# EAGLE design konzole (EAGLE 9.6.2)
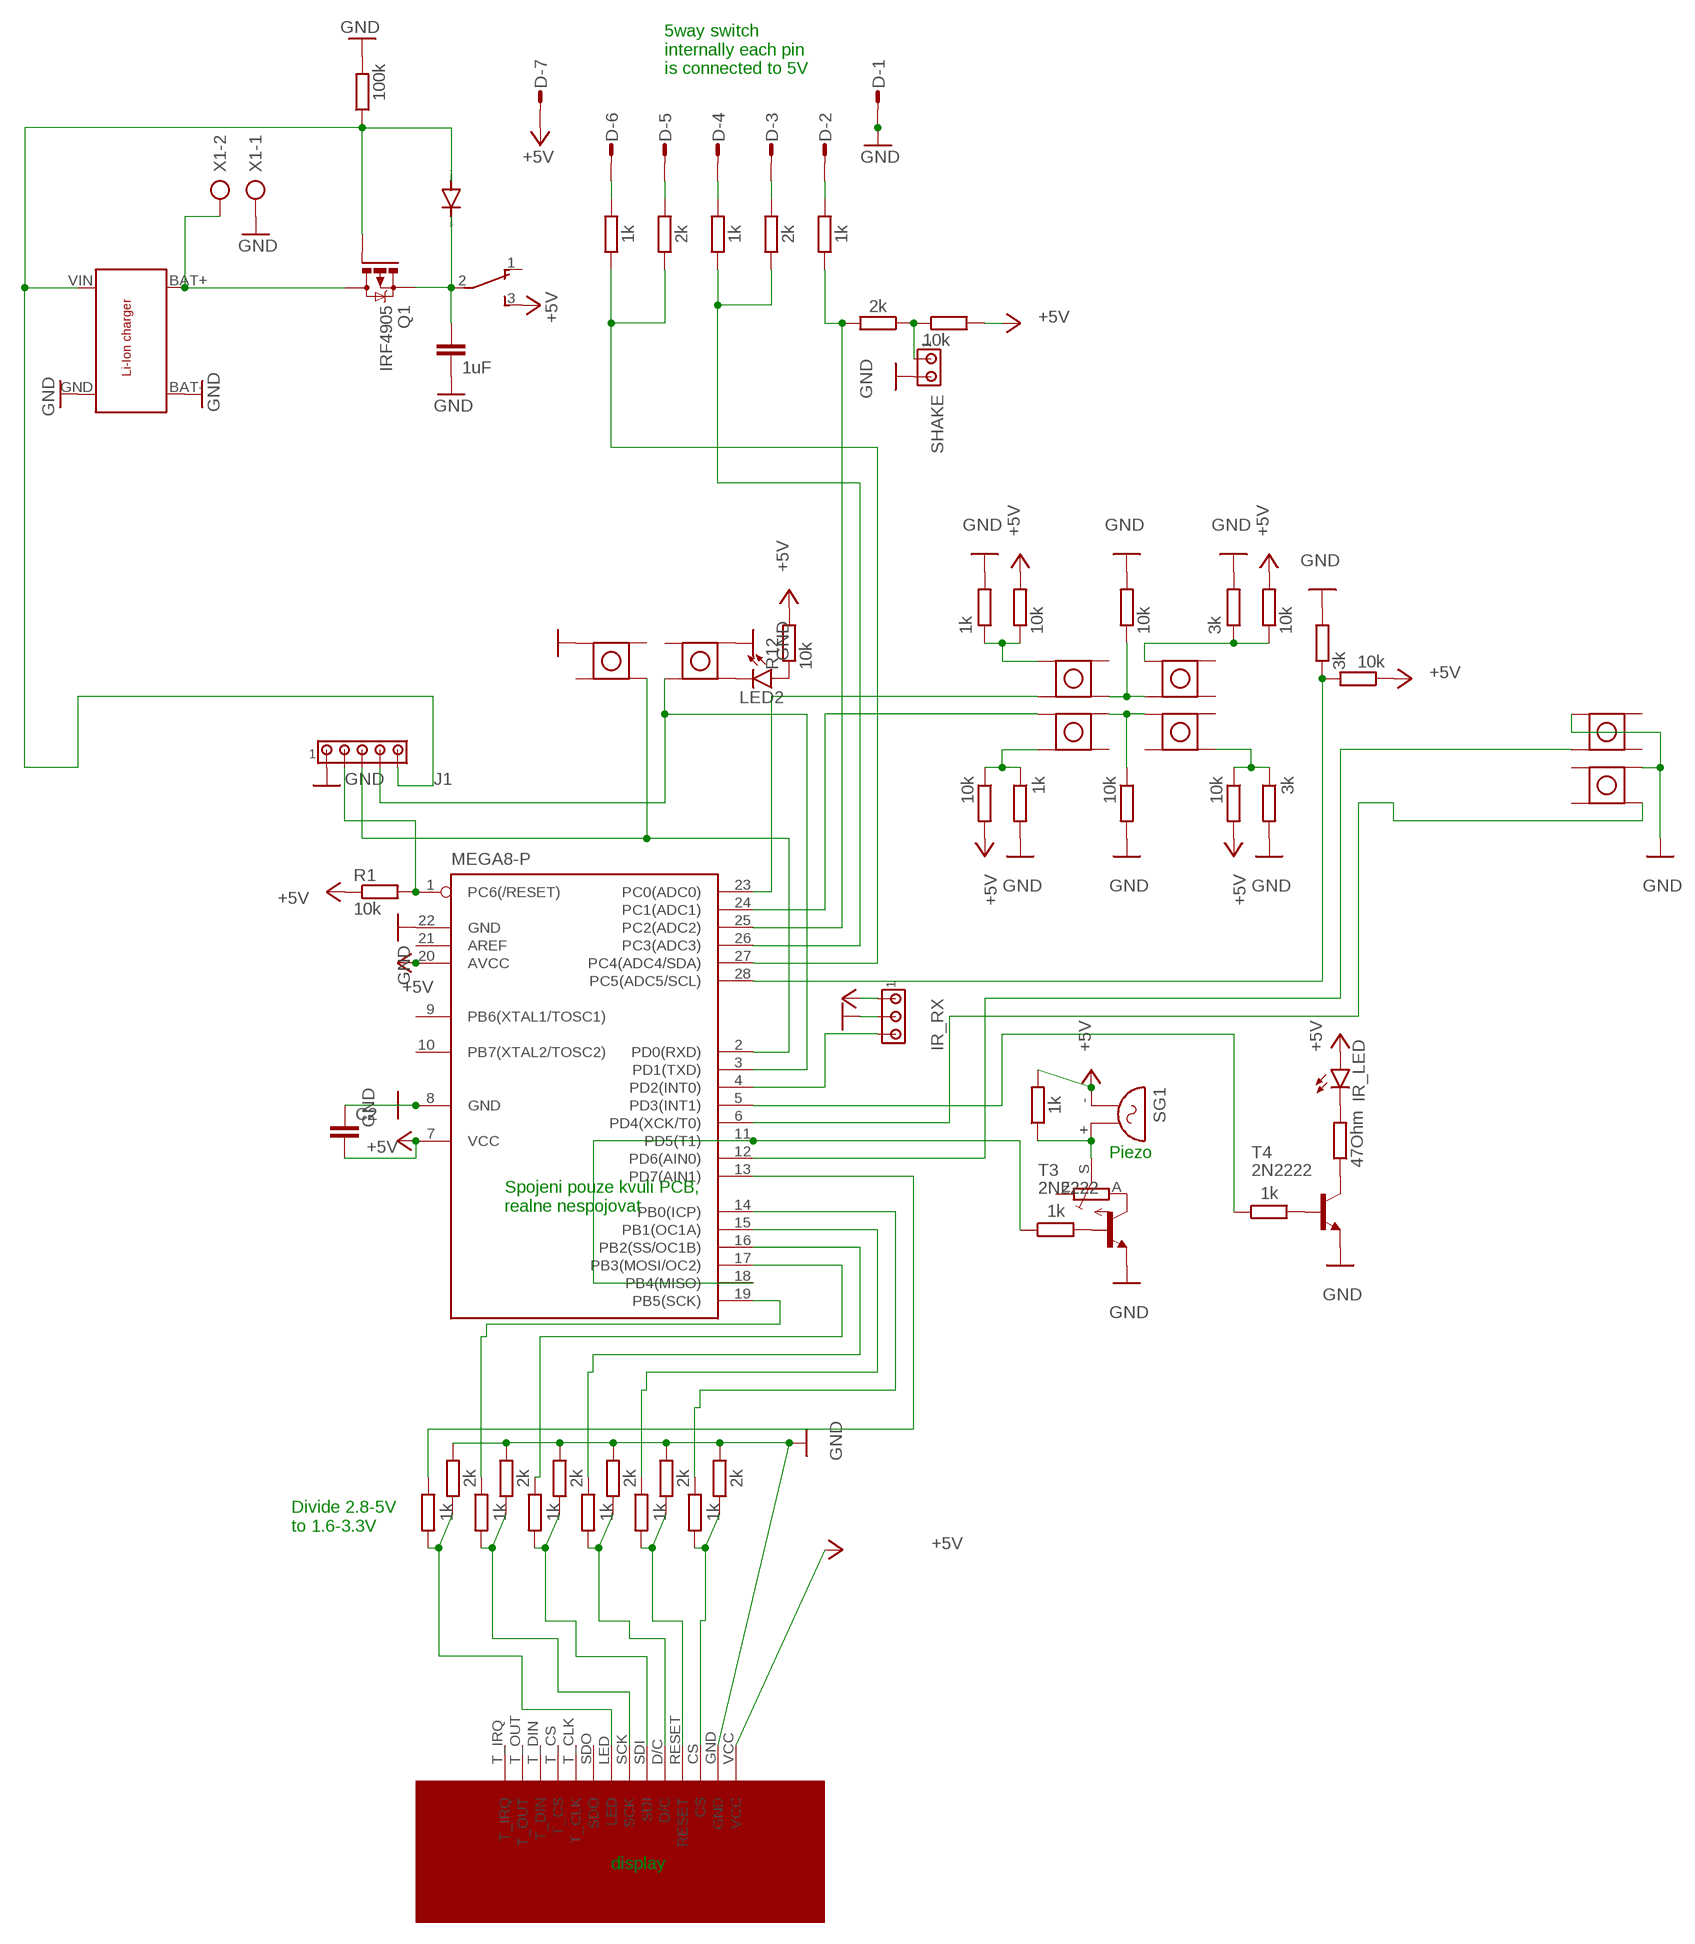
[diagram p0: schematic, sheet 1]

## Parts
C1  1uF  C-EU050-025X075  [C050-025X075]
C2  C5/2.5  [C5B2.5]
D  L07P  [L07P]
D1  1N4004  [DO41-10]
IC1  MEGA8-P  [DIL28-3]
IR_LED  LED5MM  [LED5MM]
IR_RX  MTA03-100  [10X03MTA]
J1  MTA05-100  [10X05MTA]
LED2  LED3MM  [LED3MM]
Q1  IRF4905  [TO220BH]
R1  10k  R-EU_0207/10  [0207/10]
R2  1k  R-EU_0207/10  [0207/10]
R3  2k  R-EU_0207/10  [0207/10]
R4  1k  R-EU_0207/10  [0207/10]
R5  2k  R-EU_0207/10  [0207/10]
R6  1k  R-EU_0207/10  [0207/10]
R7  2k  R-EU_0207/10  [0207/10]
R8  1k  R-EU_0207/10  [0207/10]
R9  2k  R-EU_0207/10  [0207/10]
R10  1k  R-EU_0207/10  [0207/10]
R11  2k  R-EU_0207/10  [0207/10]
R12  10k  R-EU_0207/10  [0207/10]
R13  3k  R-EU_0207/10  [0207/10]
R14  10k  R-EU_0207/10  [0207/10]
R15  1k  R-EU_0207/10  [0207/10]
R16  10k  R-EU_0207/10  [0207/10]
R17  3k  R-EU_0207/10  [0207/10]
R18  10k  R-EU_0207/10  [0207/10]
R19  1k  R-EU_0207/10  [0207/10]
R20  10k  R-EU_0207/10  [0207/10]
R21  3k  R-EU_0207/10  [0207/10]
R22  10k  R-EU_0207/10  [0207/10]
R23  10k  R-EU_0207/10  [0207/10]
R24  1k  R-EU_0207/10  [0207/10]
R25  2k  R-EU_0207/10  [0207/10]
R26  1k  R-EU_0207/10  [0207/10]
R27  1k  R-EU_0207/10  [0207/10]
R28  TRIM_EU-CIP20C-6MM  [CIP20C-6MM]
R29  10k  R-EU_0207/10  [0207/10]
R33  1k  R-EU_0207/10  [0207/10]
R34  47Ohm  R-EU_0207/10  [0207/10]
R35  1k  R-EU_0207/10  [0207/10]
R36  2k  R-EU_0207/10  [0207/10]
R38  1k  R-EU_0207/10  [0207/10]
R39  2k  R-EU_0207/10  [0207/10]
R40  1k  R-EU_0207/10  [0207/10]
R41  2k  R-EU_0207/10  [0207/10]
R42  100k  R-EU_0207/10  [0207/10]
R49  10k  R-EU_0207/10  [0207/10]
S1  TL36PO  [TL3XPO]
SG1  F/QMX  [F/QMX]
SHAKE  MTA02-100  [10X02MTA]
T3  2N2222  [TO92-EBC-OVAL]
T4  2N2222  [TO92-EBC-OVAL]
U$1  TACT  [TACT]
U$2  DISPLAY  [DISPLAY]
U$3  TACT  [TACT]
U$4  TACT  [TACT]
U$5  TACT  [TACT]
U$6  TACT  [TACT]
U$7  TACT  [TACT]
U$8  TACT  [TACT]
U$9  TACT  [TACT]
U$10  LI_ION_CHARGER  [LI_ION_CHARGER]
X1  AK500/2  [AK500/2]

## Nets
+5V: C2.2 D.7 IC1.7(VCC) IC1.20(AVCC) IR_LED.A IR_RX.1 R1.1 R12.2 R14.2 R16.2 R18.2 R20.2 R27.2 R29.1 R49.2 S1.3(S) SG1.- U$2.VCC
GND: C1.2 C2.1 D.1 IC1.8(GND) IC1.22(GND) IR_RX.2 J1.1 R3.2 R5.2 R7.2 R9.2 R11.2 R13.2 R15.2 R17.2 R19.2 R21.2 R22.2 R23.2 R25.2 R42.2 SHAKE.2 T3.E T4.E U$2.GND U$6.P$4 U$7.P$1 U$8.P$1 U$9.P$4 U$10.BAT- U$10.GND X1.1
N$1: IC1.1(PC6(/RESET)) J1.2 R1.2
N$2: R2.2 R3.1 U$2.CS
N$3: R4.2 R5.1 U$2.RESET
N$4: R6.2 R7.1 U$2.D/C
N$5: R8.2 R9.1 U$2.SDI
N$6: R10.2 R11.1 U$2.SCK
N$7: IC1.17(PB3(MOSI/OC2)) R8.1
N$8: IC1.13(PD7(AIN1)) R24.1
N$9: IC1.16(PB2(SS/OC1B)) R6.1
N$10: IC1.15(PB1(OC1A)) R4.1
N$11: R14.1 R15.1 U$1.P$1
N$12: R27.1 R28.S SG1.+
N$13: IC1.19(PB5(SCK)) R10.1
N$14: R16.1 R17.1 U$5.P$1
N$15: R18.1 R19.1 U$3.P$2
N$16: R20.1 R21.1 U$4.P$3
N$17: R33.2 T4.B
N$18: LED2.K(C) U$9.P$3
N$19: IC1.2(PD0(RXD)) J1.3 U$8.P$3
N$20: IC1.3(PD1(TXD)) J1.4 U$9.P$2
N$21: R23.1 U$3.P$4 U$4.P$1
N$22: R22.1 U$1.P$3 U$5.P$2
N$23: IC1.23(PC0(ADC0)) U$1.P$2
N$24: R24.2 R25.1 U$2.LED
N$25: IC1.24(PC1(ADC1)) U$3.P$1
N$26: R34.1 T4.C
N$27: IC1.11(PD5(T1)) IC1.18(PB4(MISO)) R26.1
N$28: R26.2 T3.B
N$29: R28.A T3.C
N$30: IC1.14(PB0(ICP)) R2.1
N$32: IC1.12(PD6(AIN0)) U$7.P$2
N$33: IC1.28(PC5(ADC5/SCL)) R13.1 R29.2
N$34: IC1.6(PD4(XCK/T0)) U$6.P$3
N$35: LED2.A R12.1
N$36: IC1.4(PD2(INT0)) IR_RX.3
N$39: IR_LED.K(C) R34.2
N$40: IC1.5(PD3(INT1)) R33.1
N$41: D.6 R38.2
N$42: D.5 R36.2
N$43: D.4 R35.2
N$44: Q1.D U$10.BAT+ X1.2
N$45: D.3 R39.2
N$46: D.2 R40.2
N$48: IC1.26(PC3(ADC3)) R35.1 R39.1
N$49: R41.1 R49.1 SHAKE.1
N$50: D1.A J1.5 Q1.G R42.1 U$10.VIN
N$51: C1.1 D1.C Q1.S S1.2(P)
N$52: IC1.25(PC2(ADC2)) R40.1 R41.2
N$54: IC1.27(PC4(ADC4/SDA)) R36.1 R38.1
Unconnected: IC1.9(PB6(XTAL1/TOSC1)) IC1.10(PB7(XTAL2/TOSC2)) IC1.21(AREF) R28.E S1.1(O) U$1.P$4 U$2.SDO U$2.T_CLK U$2.T_CS U$2.T_DIN U$2.T_IRQ U$2.T_OUT U$3.P$3 U$4.P$2 U$4.P$4 U$5.P$3 U$5.P$4 U$6.P$1 U$6.P$2 U$7.P$3 U$7.P$4 U$8.P$2 U$8.P$4 U$9.P$1

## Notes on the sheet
- 5way switch
  internally each pin
  is connected to 5V
- Piezo
- Spojeni pouze kvuli PCB, 
  realne nespojovat
- Divide 2.8-5V
  to 1.6-3.3V
- display

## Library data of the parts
C1 = rcl:C-EU: CAPACITOR, European symbol; SPICEPREFIX: C
C2 = capacitor-wima:C: CAPACITOR
D = con-amp-mt:L07P: AMP MT CONNECTOR; OC_FARNELL: unknown; OC_NEWARK: unknown
D1 = diode:1N4004: DIODE
IC1 = atmel:MEGA8-P: MICROCONTROLLER 8 Kbytes FLASH, 1 kbytes SRAM, 512 bytes EEPROM, USART, 4-channel 10 bit ADC, 2-channel 8 bit ADC Pin compatible with Atmega48, ATMega88, ATMega168 Source: avr.lbr; OC_FARNELL: unknown; OC_NEWARK: unknown
IR_LED LED2 = led:LED: LED
IR_RX = con-amp:MTA03-100: AMP connector
J1 = con-amp:MTA05-100: AMP connector
Q1 = transistor-power:IRF4905: P-Channel HEXFET® Power MOSFET RDS(on)= 0.02 Ohm, ID = -74A Source: http://www.irf.com/product-info/datasheets/data/irf4905pbf.pdf
R1-R27 R29 R33-R36 R38-R42 R49 = rcl:R-EU_: RESISTOR, European symbol; SPICEPREFIX: R
R28 = pot:TRIM_EU-: POTENTIOMETER
S1 = switch:TL36PO: TINY SWITCH ON - ON Source: http://www2.produktinfo.conrad.com/datenblaetter/700000-724999/705152-da-01-de-Subminiaturschalter_TL_36YO.pdf
SG1 = buzzer:F/QMX: BUZZER; OC_FARNELL: unknown; OC_NEWARK: unknown
SHAKE = con-amp:MTA02-100: AMP connector
T3 T4 = adafruit:2N2222: NPN TRANSISTOR Big oval pads
U$1 U$3-U$9 = PSicho:TACT
U$2 = PSicho:DISPLAY
U$10 = PSicho:LI_ION_CHARGER
X1 = con-ptr500:AK500/2: CONNECTOR; OC_FARNELL: unknown; OC_NEWARK: unknown

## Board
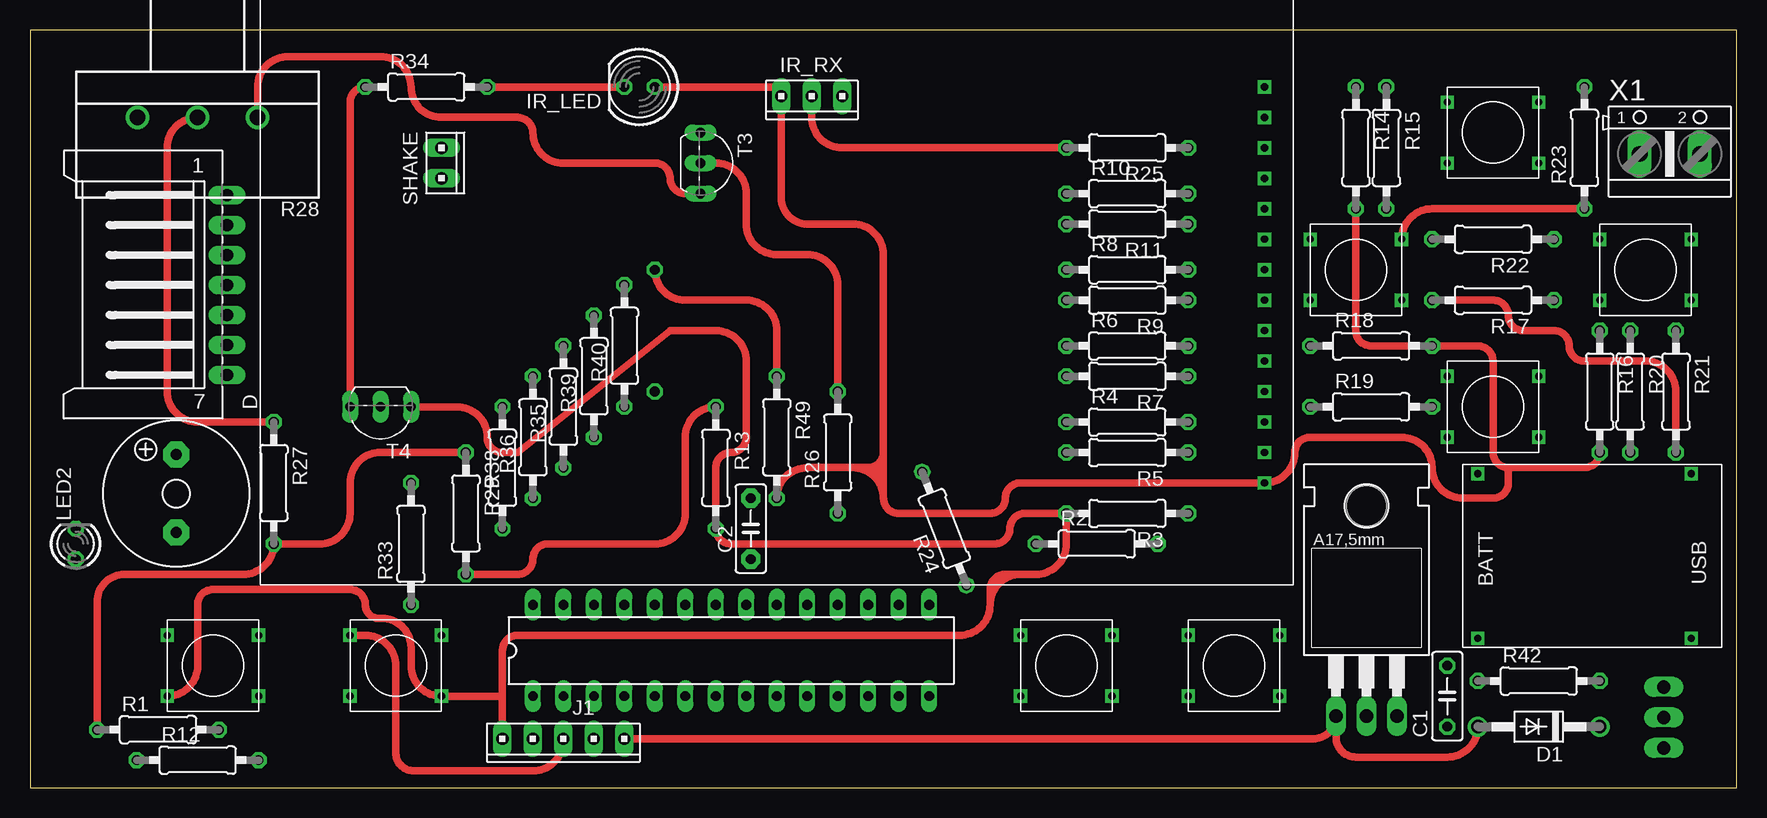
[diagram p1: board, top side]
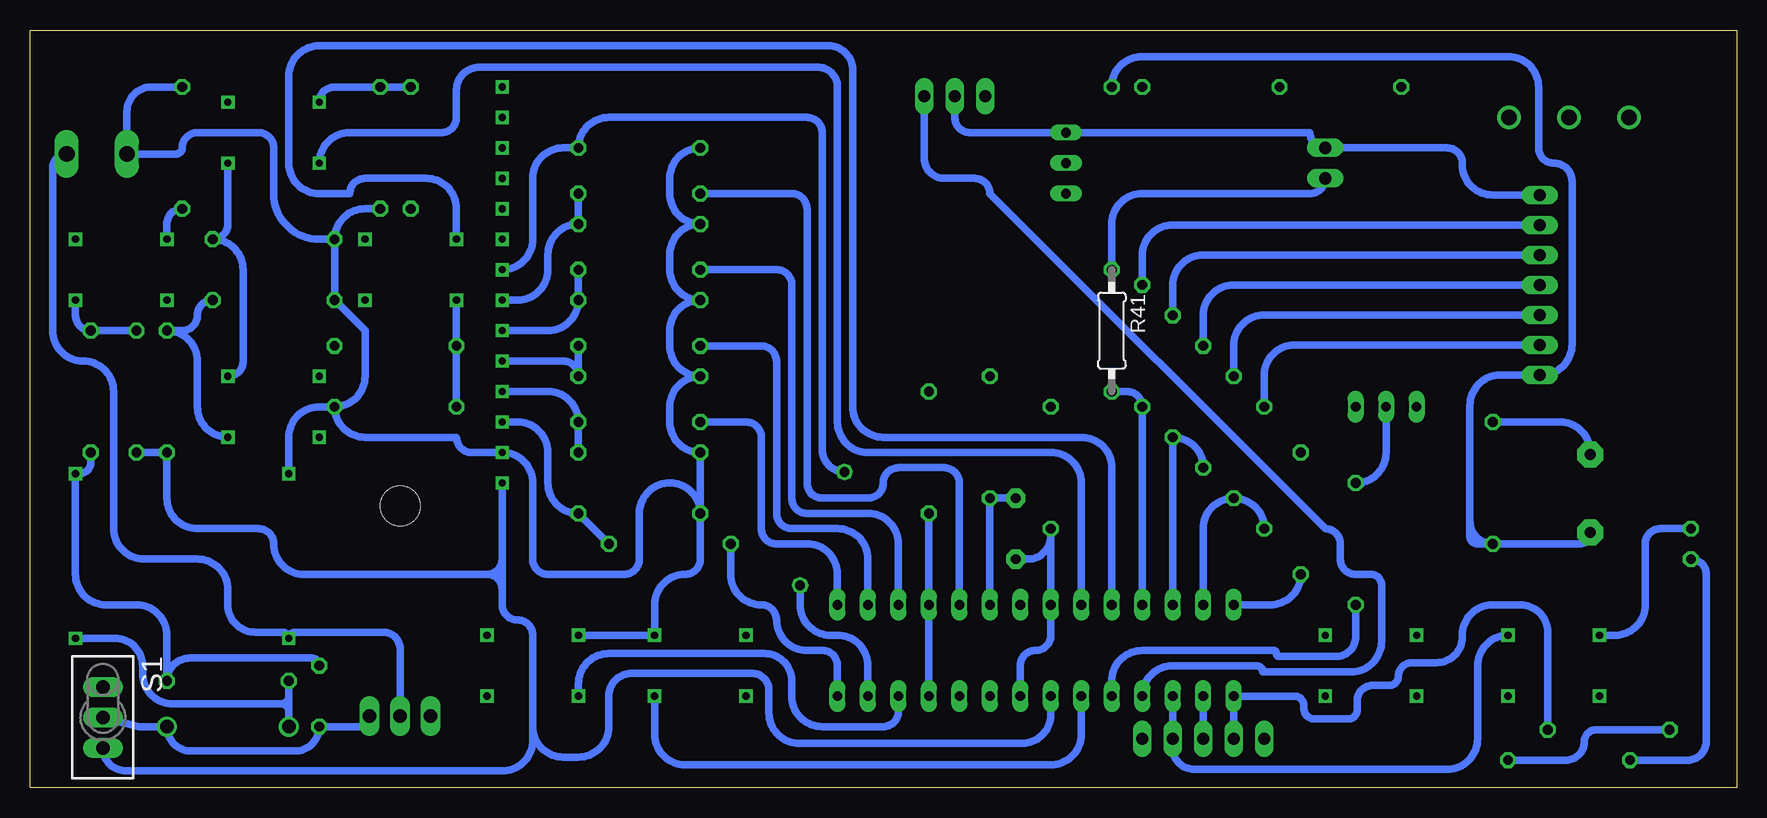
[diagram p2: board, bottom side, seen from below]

Size 142.22 x 63.17 mm. Coordinates in mm from the lower left corner, seen from the top.
Outline: 0,0 142.22,0 142.22,63.17 0,63.17 0,0
Copper layers (1*16): Top 0.035mm / dielectric 1.5mm / Bottom 0.035mm
Design rules "default *": minimum track width 24mil, minimum drill 0.6mm, track to track 24mil, track to pad 24mil, pad to pad 24mil, via to via 24mil, smd to smd 6mil, copper to edge 40mil, drill to drill 6mil, minimum pad ring 10mil, minimum via ring 8mil, stop-mask expansion 4mil, vias tented up to drill 0mil, thermal gap 10mil

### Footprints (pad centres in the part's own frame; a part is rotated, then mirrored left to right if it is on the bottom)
C050-025X075 = drill 0.813 octagon: 1 -2.54,0; 2 2.54,0
C5B2.5 = drill 0.813 pad 1.6 octagon: 1 -2.54,0; 2 2.54,0
L07P = drill 1.016 long: 1 7.5,-6.25; 2 5,-6.25; 3 2.5,-6.25; 4 0,-6.25; 5 -2.5,-6.25; 6 -5,-6.25; 7 -7.5,-6.25
DO41-10 = drill 1.118: A 5.08,0; C -5.08,0
DIL28-3 = drill 0.813 long: 1 -16.51,-3.81; 2 -13.97,-3.81; 3 -11.43,-3.81; 4 -8.89,-3.81; 5 -6.35,-3.81; 6 -3.81,-3.81; 7 -1.27,-3.81; 8 1.27,-3.81; 9 3.81,-3.81; 10 6.35,-3.81; 11 8.89,-3.81; 12 11.43,-3.81; 13 13.97,-3.81; 14 16.51,-3.81; 15 16.51,3.81; 16 13.97,3.81; 17 11.43,3.81; 18 8.89,3.81; 19 6.35,3.81; 20 3.81,3.81; 21 1.27,3.81; 22 -1.27,3.81; 23 -3.81,3.81; 24 -6.35,3.81; 25 -8.89,3.81; 26 -11.43,3.81; 27 -13.97,3.81; 28 -16.51,3.81
LED5MM = drill 0.813 octagon: A -1.27,0; K 1.27,0
10X03MTA = drill 1.016 long: 1 2.54,0; 2 0,0; 3 -2.54,0
10X05MTA = drill 1.016 long: 1 5.08,0; 2 2.54,0; 3 0,0; 4 -2.54,0; 5 -5.08,0
LED3MM = drill 0.813 octagon: A -1.27,0; K 1.27,0
TO220BH = drill 1.118 long: D 0,-6.35; G -2.54,-6.35; S 2.54,-6.35 | hole 3.302: 0,11.176
0207/10 = drill 0.813 octagon: 1 -5.08,0; 2 5.08,0
CIP20C-6MM = drill 1.3 pad 1.93: A -5,0; E 5,0; S 0,0
TL3XPO = drill 1.1 pad 1.422 long: 1 -2.54,0; 2 0,0; 3 2.54,0
F/QMX = drill 0.914 pad 2.159 octagon: + 3.251,0; - -3.251,0
10X02MTA = drill 1.016 long: 1 1.27,0; 2 -1.27,0
TO92-EBC-OVAL = drill 0.813 long: B 0,-1.27; C 2.54,-1.27; E -2.54,-1.27
TACT = drill 0.6 square: P$1 -3.81,2.54; P$2 -3.81,-2.54; P$3 3.81,-2.54; P$4 3.81,2.54
DISPLAY = drill 0.6 square: CS -40.64,11.43; D/C -40.64,6.35; GND -40.64,13.97; LED -40.64,-1.27; RESET -40.64,8.89; SCK -40.64,1.27; SDI -40.64,3.81; SDO -40.64,-3.81; T_CLK -40.64,-6.35; T_CS -40.64,-8.89; T_DIN -40.64,-11.43; T_IRQ -40.64,-16.51; T_OUT -40.64,-13.97; VCC -40.64,16.51
LI_ION_CHARGER = drill 0.6 square: BAT+ 8.89,6.858; BAT- 8.89,-6.858; GND -8.89,-6.858; VIN -8.89,6.858
AK500/2 = drill 1.321 long: 1 -2.515,0; 2 2.515,0

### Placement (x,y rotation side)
C1  118.11,7.62 90 top
C2  60.07,21.59 90 top
D  10.16,41.91 90 top
D1  125.73,5.08 180 top
IC1  58.42,11.43 0 top
IR_LED  50.8,58.42 180 top
IR_RX  65.15,57.66 180 top
J1  44.45,4.06 180 top
LED2  3.81,20.32 90 top
Q1  111.38,12.32 0 top
R1  10.67,4.83 0 top
R2  88.9,20.32 0 top
R3  91.44,22.86 180 top
R4  91.44,30.48 0 top
R5  91.44,27.94 180 top
R6  91.44,36.83 0 top
R7  91.44,34.29 180 top
R8  91.44,43.18 0 top
R9  91.44,40.64 180 top
R10  91.44,49.53 0 top
R11  91.44,46.99 180 top
R12  13.97,2.29 0 top
R13  57.15,26.67 270 top
R14  110.49,53.34 270 top
R15  113.03,53.34 270 top
R16  130.81,33.02 270 top
R17  121.92,40.64 180 top
R18  111.76,36.83 0 top
R19  111.76,31.75 0 top
R20  133.35,33.02 270 top
R21  137.16,33.02 270 top
R22  121.92,45.72 180 top
R23  129.54,53.34 90 top
R24  76.2,21.59 111.3 top
R25  91.44,53.34 180 top
R26  67.31,27.94 90 top
R27  20.32,25.4 270 top
R28  13.97,55.88 180 top
R29  36.32,22.86 270 top
R33  31.75,20.32 90 top
R34  33.02,58.42 0 top
R35  44.45,31.75 90 top
R36  41.91,29.21 90 top
R38  39.37,26.67 90 top
R39  46.99,34.29 90 top
R40  49.53,36.83 90 top
R41  52.07,38.1 270 bottom
R42  125.73,8.89 0 top
R49  62.23,29.21 270 top
S1  136.14,5.84 270 bottom
SG1  12.19,24.51 90 top
SHAKE  34.29,52.07 270 top
T3  57.15,52.07 270 top
T4  29.21,30.48 180 top
U$1  121.92,54.61 0 top
U$2  62.23,41.91 180 top
U$3  110.49,43.18 0 top
U$4  134.62,43.18 0 top
U$5  121.92,31.75 180 top
U$6  86.36,10.16 0 top
U$7  100.33,10.16 0 top
U$8  30.48,10.16 180 top
U$9  15.24,10.16 180 top
U$10  129.54,19.3 180 top
X1  136.65,52.83 0 top

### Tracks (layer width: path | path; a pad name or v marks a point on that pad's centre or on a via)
+5V
  Top 0.61: R14.2 110.49,38.1 arc90 111.76,36.83 R18.2 120.65,36.83 arc-90 121.92,35.56 121.92,27.94 arc90 123.19,26.67 | 71.12,24.13 arc90 72.39,22.86 80.01,22.86 arc90 81.28,24.13 arc-90 82.55,25.4 U$2.VCC arc90 105.41,27.94 arc-90 106.68,29.21 114.3,29.21 arc-90 116.84,26.67 arc90 119.38,24.13 121.92,24.13 arc90 123.19,25.4 123.19,26.67 | 71.12,24.13 arc90 68.58,26.67 | 68.58,26.67 64.77,26.67 arc90 R49.2 | 71.12,27.94 71.12,44.45 arc90 68.58,46.99 64.77,46.99 arc-90 62.61,49.15 IR_RX.1 arc90 61.85,58.42 IR_LED.A | 71.12,27.94 71.12,26.67 | 71.12,26.67 71.12,25.4 | 71.12,25.4 71.12,24.13 | 68.58,26.67 69.85,26.67 | 69.85,26.67 arc90 71.12,27.94 | 69.85,26.67 arc-90 71.12,25.4 | 69.85,26.67 arc90 71.12,27.94 | 69.85,26.67 71.12,26.67 | R16.2 arc-90 129.54,26.67 123.19,26.67 | R1.1 5.59,15.49 arc-90 7.87,17.78 17.78,17.78 arc90 R27.2 24.13,20.32 arc90 26.67,22.86 26.67,25.4 arc-90 29.21,27.94 R29.1
  Bottom 0.61: 100.33,5.08 100.33,12.7 arc-90 101.6,13.97 arc90 102.87,15.24 102.87,16.51 | 102.87,16.51 102.87,17.78 | 102.87,17.78 102.87,19.05 | 102.87,19.05 U$2.VCC | IC1.7 57.15,6.1 arc90 59.56,3.68 78.1,3.68 arc90 80.65,6.22 80.65,8.13 arc-90 82.04,9.52 92.07,9.52 arc-90 93.98,7.62 93.98,5.08 arc90 96.52,2.54 97.79,2.54 arc90 100.33,5.08 | R20.2 R16.2 130.81,24.13 arc-90 128.27,21.59 123.19,21.59 arc90 121.92,20.32 arc-90 119.38,17.78 104.14,17.78 | R27.2 13.13,20.32 arc-90 SG1.- | R27.2 21.59,20.32 arc90 22.23,20.95 22.23,22.23 | 22.23,22.23 arc-90 R27.2 | 22.23,22.23 22.23,31.87 arc90 19.69,34.41 D.7 16.26,34.41 arc-90 13.72,36.95 13.72,50.55 arc-90 15.24,52.07 arc90 16.51,53.34 16.51,58.42 arc-90 19.05,60.96 49.53,60.96 arc-90 IR_LED.A | S1.3 arc-90 134.24,1.4 102.87,1.4 arc-90 100.33,3.94 100.33,5.08 | R12.2 14.22,2.29 arc-90 12.7,3.81 arc90 11.68,4.83 R1.1 | IC1.20 R49.2 C2.2 | 102.87,17.78 104.14,17.78 | 104.14,17.78 arc-90 102.87,19.05 | 104.14,17.78 arc90 102.87,16.51
GND
  Top 0.61: R21.2 137.16,33.02 arc90 134.62,35.56 129.54,35.56 arc-90 128.27,36.83 arc90 127,38.1 124.46,38.1 arc-90 123.19,39.37 arc90 121.92,40.64 R17.2 | 82.55,17.78 81.28,17.78 arc90 80.01,16.51 80.01,15.24 | 82.55,17.78 arc90 80.01,15.24 | 80.01,15.24 arc-90 77.47,12.7 40.64,12.7 arc90 39.37,11.43 39.37,7.62 | 39.37,7.62 J1.1 | R25.2 67.69,53.34 arc-90 65.15,55.88 IR_RX.2 | 82.55,17.78 83.82,17.78 arc90 86.36,20.32 R3.2 82.93,22.86 arc90 81.66,21.59 arc-90 80.39,20.32 58.42,20.32 arc-90 R13.2 57.15,26.67 arc-90 58.42,27.94 arc90 59.69,29.21 59.69,35.56 arc90 57.15,38.1 53.34,38.1 40.64,27.94 39.37,27.94 arc-90 38.1,29.21 arc90 35.56,31.75 T4.E | 39.37,7.62 U$8.P$1 arc-90 31.75,10.16 31.75,11.68 arc90 29.34,14.1 29.08,14.1 arc-90 27.94,15.24 arc90 26.67,16.51 15.24,16.51 arc90 13.97,15.24 13.97,10.16 arc-90 U$9.P$4
  Bottom 0.61: R3.2 arc-90 88.9,25.4 arc-90 91.44,22.86 91.44,19.05 arc90 92.71,17.78 99.06,17.78 arc90 100.33,19.05 100.33,25.4 arc-90 U$2.GND 105.41,27.94 arc90 106.68,29.21 114.3,29.21 arc90 R19.2 | R3.2 R5.2 arc90 88.9,30.48 88.9,31.75 arc90 R7.2 arc90 88.9,36.83 88.9,38.1 arc90 R9.2 arc90 88.9,43.18 88.9,44.45 arc90 R11.2 arc90 88.9,49.53 88.9,50.8 arc90 R25.2 | R23.2 132.08,58.42 arc-90 134.14,56.36 X1.1 130.05,52.83 arc-90 129.54,53.34 arc90 128.27,54.61 123.19,54.61 arc90 121.92,53.34 121.92,49.53 arc-90 118.11,45.72 R22.2 | R22.2 R17.2 114.3,38.1 114.3,34.29 arc90 R19.2 | R22.2 arc90 114.3,48.26 R15.2 | U$6.P$4 U$7.P$1 94.23,12.7 | U$6.P$4 90.17,15.24 arc90 87.63,17.78 arc-90 86.36,19.05 R3.2 | IC1.8 59.69,10.16 arc90 58.42,11.43 arc-90 57.15,12.7 IC1.22 R13.2 57.15,20.95 arc90 59.05,19.05 C2.1 | IR_RX.2 65.15,55.88 arc-90 63.88,54.61 T3.E 35.56,54.61 arc-90 SHAKE.2 24.13,53.34 arc90 22.86,52.07 22.86,51.95 arc-90 20.32,49.41 D.1 | R21.2 137.16,26.92 arc90 U$10.GND 138.43,17.78 arc-90 135.89,15.24 133.35,15.24 arc90 130.81,12.7 R42.2 arc90 128.91,10.8 118.75,10.8 arc90 C1.2 | R19.2 118.11,31.75 arc-90 120.65,29.21 U$10.BAT- | U$6.P$4 92.46,12.7
N$1
  Bottom 0.61: J1.2 IC1.1 36.83,7.62 arc90 36.07,6.86 36.07,6.6 arc-90 35.18,5.71 32.38,5.71 arc-90 31.62,6.48 31.62,7.24 arc90 30.35,8.51 28.96,8.51 arc-90 28.19,9.27 arc90 27.05,10.41 25.02,10.41 arc-90 22.86,12.57 22.86,12.7 arc90 20.32,15.24 18.03,15.24 arc90 15.75,12.95 R1.2
N$2
  Bottom 0.61: R2.2 R3.1 arc90 99.06,25.4 99.06,27.94 arc-90 101.6,30.48 U$2.CS
N$3
  Bottom 0.61: R5.1 R4.2 arc-90 99.06,33.02 U$2.RESET
N$4
  Bottom 0.61: R6.2 R7.1 arc-90 97.79,35.56 U$2.D/C
N$5
  Bottom 0.61: R8.2 R9.1 arc90 99.06,38.1 U$2.SDI
N$6
  Bottom 0.61: U$2.SCK 101.6,40.64 arc-90 99.06,43.18 99.06,44.45 arc90 R11.1 R10.2
N$7
  Bottom 0.61: IC1.17 69.85,20.32 arc-90 72.39,22.86 77.47,22.86 arc90 78.74,24.13 78.74,41.91 arc-90 80.01,43.18 R8.1
N$8
  Bottom 0.61: R24.1 78.04,15.24 arc-90 75.5,12.7 74.93,12.7 arc90 72.39,10.16 IC1.13
N$9
  Bottom 0.61: IC1.16 72.39,19.05 arc-90 74.93,21.59 78.74,21.59 arc90 80.01,22.86 80.01,35.56 arc-90 81.28,36.83 R6.1
N$10
  Bottom 0.61: IC1.15 74.93,17.78 arc-90 77.47,20.32 80.01,20.32 arc90 81.28,21.59 81.28,29.21 arc-90 82.55,30.48 R4.1
N$11
  Bottom 0.61: R14.1 R15.1 116.84,58.42 arc-90 U$1.P$1
N$12
  Top 0.61: R27.1 13.97,30.48 arc-90 11.43,33.02 11.43,53.34 arc-90 R28.S
  Bottom 0.61: R27.1 14.73,30.48 arc90 12.19,27.94 SG1.+
N$13
  Bottom 0.61: R10.1 78.74,49.53 arc90 77.47,48.26 77.47,25.4 arc-90 76.2,24.13 72.39,24.13 arc-90 71.12,25.4 arc90 69.85,26.67 66.04,26.67 arc90 64.77,25.4 IC1.19
N$14
  Bottom 0.61: U$5.P$1 arc90 128.27,31.75 128.27,35.56 arc-90 R16.1 129.54,38.1 arc-90 128.27,39.37 arc90 R17.1
N$15
  Bottom 0.61: U$3.P$2 R18.1 R19.1
N$16
  Bottom 0.61: R20.1 R21.1 arc90 138.43,39.37 U$4.P$3
N$17
  Bottom 0.61: R33.2 arc-90 29.21,27.94 T4.B
N$18
  Bottom 0.61: U$9.P$3 10.16,12.7 arc-90 7.62,15.24 7.62,20.32 arc90 6.35,21.59 LED2.K
N$19
  Top 0.61: U$8.P$3 27.94,12.7 arc-90 30.48,10.16 30.48,2.92 arc90 32,1.4 41.91,1.4 arc90 44.45,3.94 J1.3
  Bottom 0.61: IC1.2 J1.3
N$20
  Bottom 0.61: IC1.3 J1.4 46.99,3.3 arc-90 45.21,1.52 24.13,1.52 arc-90 21.59,4.06 21.59,10.16 arc90 U$9.P$2
N$21
  Top 0.61: R23.1 116.84,48.26 arc90 U$3.P$4
  Bottom 0.61: U$4.P$1 130.81,46.99 arc90 R23.1
N$22
  Bottom 0.61: U$5.P$2 arc-90 124.46,35.56 124.46,43.18 arc-90 R22.1 arc-90 125.73,46.99 U$1.P$3
N$23
  Bottom 0.61: U$1.P$2 arc90 115.57,54.61 107.95,54.61 arc-90 106.68,55.88 106.68,58.17 arc90 104.78,60.07 76.58,60.07 arc90 74.93,58.42 74.93,30.48 arc-90 72.39,27.94 57.15,27.94 arc90 54.61,25.4 IC1.23
N$24
  Bottom 0.61: U$2.LED arc-90 100.33,45.72 100.33,50.8 arc90 97.79,53.34 R25.1 arc90 93.98,55.88 77.47,55.88 arc90 76.2,54.61 76.2,28.17 arc-90 R24.2
N$25
  Bottom 0.61: IC1.24 52.07,26.67 arc-90 54.61,29.21 71.12,29.21 arc90 73.66,31.75 73.66,59.82 arc-90 75.69,61.85 118.11,61.85 arc-90 120.65,59.31 120.65,52.07 arc-90 118.11,49.53 115.57,49.53 arc90 114.3,50.8 109.22,50.8 arc90 106.68,48.26 U$3.P$1
N$26
  Top 0.61: T4.C 26.67,57.15 arc-90 R34.1
N$27
  Bottom 0.61: R26.1 IC1.18 IC1.11
N$28
  Top 0.61: R26.2 67.31,41.91 arc90 64.77,44.45 62.23,44.45 arc-90 59.69,46.99 59.69,49.53 arc90 57.15,52.07 T3.B
N$29
  Top 0.61: T3.C 54.61,49.53 arc-90 53.34,50.8 arc90 52.07,52.07 44.45,52.07 arc-90 41.91,54.61 arc90 40.64,55.88 34.29,55.88 arc-90 31.75,58.42 arc90 29.21,60.96 21.51,60.96 arc90 18.97,58.42 R28.A
N$30
  Bottom 0.61: R2.1 83.82,17.78 arc-90 81.28,15.24 arc90 80.01,13.97 arc-90 77.47,11.43 76.2,11.43 arc90 74.93,10.16 IC1.14
N$32
  Bottom 0.61: U$7.P$2 96.52,8.64 arc90 93.98,11.18 81.03,11.18 arc90 78.74,8.89 78.74,7.62 arc-90 76.2,5.08 71.12,5.08 arc-90 69.85,6.35 IC1.12
N$33
  Top 0.61: R13.1 arc90 54.61,29.21 54.61,22.86 arc-90 52.07,20.32 43.18,20.32 arc90 41.91,19.05 arc-90 40.64,17.78 R29.2
  Bottom 0.61: IC1.28 38.86,15.24 arc-90 R29.2
N$34
  Bottom 0.61: IC1.6 54.61,4.45 arc90 57.15,1.9 87.63,1.9 arc90 90.17,4.45 U$6.P$3
N$35
  Bottom 0.61: LED2.A arc90 2.54,17.78 2.54,3.81 arc90 4.06,2.29 R12.1
N$36
  Bottom 0.61: IC1.4 arc90 46.99,10.16 40.01,10.16 arc90 39.5,9.65 32.13,9.65 arc-90 29.59,12.19 29.59,16.89 arc-90 30.48,17.78 31.75,17.78 arc90 33.02,19.05 33.02,20.32 arc-90 34.29,21.59 62.23,49.53 arc-90 63.5,50.8 66.04,50.8 arc90 67.69,52.45 IR_RX.3
N$39
  Top 0.61: IR_LED.K R34.2
N$40
  Bottom 0.61: IC1.5 52.07,8.89 arc90 49.53,11.43 38.61,11.43 arc90 38.35,11.18 arc-90 38.1,10.92 33.4,10.92 arc-90 31.75,12.57 R33.1
N$41
  Bottom 0.61: R38.2 39.37,34.37 arc90 36.83,36.91 D.6
N$42
  Bottom 0.61: R36.2 41.91,36.87 arc90 39.37,39.41 D.5
N$43
  Bottom 0.61: R35.2 44.45,39.37 arc90 41.91,41.91 D.4
N$44
  Bottom 0.61: Q1.D 111.38,11.56 arc-90 112.78,12.95 120.14,12.95 arc-90 U$10.BAT+ arc-90 121.16,12.95 123.44,12.95 arc90 125.73,15.24 125.73,16.51 arc-90 128.27,19.05 132.72,19.05 arc90 135.25,21.59 135.25,33.02 arc-90 137.79,35.56 arc90 140.34,38.1 140.34,51.66 arc90 X1.2
N$45
  Bottom 0.61: R39.2 46.99,41.87 arc90 44.45,44.41 D.3
N$46
  Bottom 0.61: R40.2 49.53,44.37 arc90 46.99,46.91 D.2
N$48
  Bottom 0.61: IC1.26 R39.1 arc90 R35.1
N$49
  Top 0.61: R49.1 62.23,38.1 arc90 59.69,40.64 54.61,40.64 arc-90 R41.1
  Bottom 0.61: R41.1 52.07,46.99 arc90 49.53,49.53 35.56,49.53 arc-90 SHAKE.1
N$50
  Top 0.61: D1.A arc-90 118.11,2.54 110.49,2.54 arc-90 108.84,4.19 Q1.G arc-90 106.93,4.06 J1.5
  Bottom 0.61: R42.1 120.65,7.62 | 120.65,7.62 120.65,6.35 | 120.65,6.35 D1.A | 120.65,6.35 arc-90 121.28,6.98 | 121.28,6.98 130.3,6.98 arc90 132.84,9.52 132.84,10.16 arc-90 135.13,12.45 U$10.VIN | 121.28,6.98 arc-90 120.65,7.62
N$51
  Bottom 0.61: Q1.S arc90 114.81,5.08 C1.1 arc90 120.14,3.05 128.78,3.05 arc90 D1.C 133.1,5.08 S1.2
N$52
  Bottom 0.61: IC1.25 R40.1 arc-90 50.8,33.02 R41.2
N$54
  Bottom 0.61: IC1.27 44.45,21.59 arc90 R36.1 arc90 R38.1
